DATA_BLOCK DB_AIS
TITLE = Analog Inputs SRC
//Analog Input Source DATA Block
VERSION : 0.1
  STRUCT
K04HJA10CR001XQ01 : UAI_SRC; //HOØÁK È.1 - VELIKOST PLAMENE 4-20mA
K04HJA20CR001XQ01 : UAI_SRC; //HOØÁK È.2 - VELIKOST PLAMENE 4-20mA
K04HJA30CR001XQ01 : UAI_SRC; //HOØÁK È.3 - VELIKOST PLAMENE 4-20mA
K04HJA40CR001XQ01 : UAI_SRC; //HOØÁK È.4 - VELIKOST PLAMENE 4-20mA
K04HHG36AS001XQ01 : UAI_SRC; //HOØÁK È.1 - POLOHA KLAPKY PLYNU
K04HHL11AS010XQ01 : UAI_SRC; //HOØÁK È.1 - POLOHA KLAPKY VZDUCHU
K04HHG37AS001XQ01 : UAI_SRC; //HOØÁK È.2 - POLOHA KLAPKY PLYNU
K04HHL71AS010XQ01 : UAI_SRC; //HOØÁK È.2 - POLOHA KLAPKY VZDUCHU
K04HHG38AS001XQ01 : UAI_SRC; //HOØÁK È.3 - POLOHA KLAPKY PLYNU
K04HHL51AS010XQ01 : UAI_SRC; //HOØÁK È.3 - POLOHA KLAPKY VZDUCHU
K04HHG39AS001XQ01 : UAI_SRC; //HOØÁK È.4 - POLOHA KLAPKY PLYNU
K04HHL31AS010XQ01 : UAI_SRC; //HOØÁK È.4 - POLOHA KLAPKY VZDUCHU
PIW536 : UAI_SRC; //REZERVA
PIW538 : UAI_SRC; //REZERVA
PIW540 : UAI_SRC; //REZERVA
PIW542 : UAI_SRC; //REZERVA
END_STRUCT ;
BEGIN

K04HJA10CR001XQ01.cMEAS_TYPE := 00;
K04HJA10CR001XQ01.cENABLE_REV := FALSE;
K04HJA10CR001XQ01.cLRANGE := 0.000;
K04HJA10CR001XQ01.cHRANGE := 100.000;
K04HJA10CR001XQ01.cENABLE_SQRT := FALSE;
K04HJA10CR001XQ01.cENABLE_LOLO := False;
K04HJA10CR001XQ01.cENABLE_LO := False;
K04HJA10CR001XQ01.cENABLE_HIHI := False;
K04HJA10CR001XQ01.cENABLE_HI := False;
K04HJA10CR001XQ01.cSET_LOLO := 0.000;
K04HJA10CR001XQ01.cSET_LO := 0.000;
K04HJA10CR001XQ01.cSET_HIHI := 100.000;
K04HJA10CR001XQ01.cSET_HI := 100.000;
K04HJA20CR001XQ01.cMEAS_TYPE := 00;
K04HJA20CR001XQ01.cENABLE_REV := FALSE;
K04HJA20CR001XQ01.cLRANGE := 0.000;
K04HJA20CR001XQ01.cHRANGE := 100.000;
K04HJA20CR001XQ01.cENABLE_SQRT := FALSE;
K04HJA20CR001XQ01.cENABLE_LOLO := False;
K04HJA20CR001XQ01.cENABLE_LO := False;
K04HJA20CR001XQ01.cENABLE_HIHI := False;
K04HJA20CR001XQ01.cENABLE_HI := False;
K04HJA20CR001XQ01.cSET_LOLO := 0.000;
K04HJA20CR001XQ01.cSET_LO := 0.000;
K04HJA20CR001XQ01.cSET_HIHI := 100.000;
K04HJA20CR001XQ01.cSET_HI := 100.000;
K04HJA30CR001XQ01.cMEAS_TYPE := 00;
K04HJA30CR001XQ01.cENABLE_REV := FALSE;
K04HJA30CR001XQ01.cLRANGE := 0.000;
K04HJA30CR001XQ01.cHRANGE := 100.000;
K04HJA30CR001XQ01.cENABLE_SQRT := FALSE;
K04HJA30CR001XQ01.cENABLE_LOLO := False;
K04HJA30CR001XQ01.cENABLE_LO := False;
K04HJA30CR001XQ01.cENABLE_HIHI := False;
K04HJA30CR001XQ01.cENABLE_HI := False;
K04HJA30CR001XQ01.cSET_LOLO := 0.000;
K04HJA30CR001XQ01.cSET_LO := 0.000;
K04HJA30CR001XQ01.cSET_HIHI := 100.000;
K04HJA30CR001XQ01.cSET_HI := 100.000;
K04HJA40CR001XQ01.cMEAS_TYPE := 00;
K04HJA40CR001XQ01.cENABLE_REV := FALSE;
K04HJA40CR001XQ01.cLRANGE := 0.000;
K04HJA40CR001XQ01.cHRANGE := 100.000;
K04HJA40CR001XQ01.cENABLE_SQRT := FALSE;
K04HJA40CR001XQ01.cENABLE_LOLO := False;
K04HJA40CR001XQ01.cENABLE_LO := False;
K04HJA40CR001XQ01.cENABLE_HIHI := False;
K04HJA40CR001XQ01.cENABLE_HI := False;
K04HJA40CR001XQ01.cSET_LOLO := 0.000;
K04HJA40CR001XQ01.cSET_LO := 0.000;
K04HJA40CR001XQ01.cSET_HIHI := 100.000;
K04HJA40CR001XQ01.cSET_HI := 100.000;
K04HHG36AS001XQ01.cMEAS_TYPE := 00;
K04HHG36AS001XQ01.cENABLE_REV := FALSE;
K04HHG36AS001XQ01.cLRANGE := 0.000;
K04HHG36AS001XQ01.cHRANGE := 100.000;
K04HHG36AS001XQ01.cENABLE_SQRT := FALSE;
K04HHG36AS001XQ01.cENABLE_LOLO := False;
K04HHG36AS001XQ01.cENABLE_LO := False;
K04HHG36AS001XQ01.cENABLE_HIHI := False;
K04HHG36AS001XQ01.cENABLE_HI := False;
K04HHG36AS001XQ01.cSET_LOLO := 0.000;
K04HHG36AS001XQ01.cSET_LO := 0.000;
K04HHG36AS001XQ01.cSET_HIHI := 100.000;
K04HHG36AS001XQ01.cSET_HI := 100.000;
K04HHL11AS010XQ01.cMEAS_TYPE := 00;
K04HHL11AS010XQ01.cENABLE_REV := FALSE;
K04HHL11AS010XQ01.cLRANGE := 0.000;
K04HHL11AS010XQ01.cHRANGE := 100.000;
K04HHL11AS010XQ01.cENABLE_SQRT := FALSE;
K04HHL11AS010XQ01.cENABLE_LOLO := False;
K04HHL11AS010XQ01.cENABLE_LO := False;
K04HHL11AS010XQ01.cENABLE_HIHI := False;
K04HHL11AS010XQ01.cENABLE_HI := False;
K04HHL11AS010XQ01.cSET_LOLO := 0.000;
K04HHL11AS010XQ01.cSET_LO := 0.000;
K04HHL11AS010XQ01.cSET_HIHI := 100.000;
K04HHL11AS010XQ01.cSET_HI := 100.000;
K04HHG37AS001XQ01.cMEAS_TYPE := 00;
K04HHG37AS001XQ01.cENABLE_REV := FALSE;
K04HHG37AS001XQ01.cLRANGE := 0.000;
K04HHG37AS001XQ01.cHRANGE := 100.000;
K04HHG37AS001XQ01.cENABLE_SQRT := FALSE;
K04HHG37AS001XQ01.cENABLE_LOLO := False;
K04HHG37AS001XQ01.cENABLE_LO := False;
K04HHG37AS001XQ01.cENABLE_HIHI := False;
K04HHG37AS001XQ01.cENABLE_HI := False;
K04HHG37AS001XQ01.cSET_LOLO := 0.000;
K04HHG37AS001XQ01.cSET_LO := 0.000;
K04HHG37AS001XQ01.cSET_HIHI := 100.000;
K04HHG37AS001XQ01.cSET_HI := 100.000;
K04HHL71AS010XQ01.cMEAS_TYPE := 00;
K04HHL71AS010XQ01.cENABLE_REV := FALSE;
K04HHL71AS010XQ01.cLRANGE := 0.000;
K04HHL71AS010XQ01.cHRANGE := 100.000;
K04HHL71AS010XQ01.cENABLE_SQRT := FALSE;
K04HHL71AS010XQ01.cENABLE_LOLO := False;
K04HHL71AS010XQ01.cENABLE_LO := False;
K04HHL71AS010XQ01.cENABLE_HIHI := False;
K04HHL71AS010XQ01.cENABLE_HI := False;
K04HHL71AS010XQ01.cSET_LOLO := 0.000;
K04HHL71AS010XQ01.cSET_LO := 0.000;
K04HHL71AS010XQ01.cSET_HIHI := 100.000;
K04HHL71AS010XQ01.cSET_HI := 100.000;
K04HHG38AS001XQ01.cMEAS_TYPE := 00;
K04HHG38AS001XQ01.cENABLE_REV := FALSE;
K04HHG38AS001XQ01.cLRANGE := 0.000;
K04HHG38AS001XQ01.cHRANGE := 100.000;
K04HHG38AS001XQ01.cENABLE_SQRT := FALSE;
K04HHG38AS001XQ01.cENABLE_LOLO := False;
K04HHG38AS001XQ01.cENABLE_LO := False;
K04HHG38AS001XQ01.cENABLE_HIHI := False;
K04HHG38AS001XQ01.cENABLE_HI := False;
K04HHG38AS001XQ01.cSET_LOLO := 0.000;
K04HHG38AS001XQ01.cSET_LO := 0.000;
K04HHG38AS001XQ01.cSET_HIHI := 100.000;
K04HHG38AS001XQ01.cSET_HI := 100.000;
K04HHL51AS010XQ01.cMEAS_TYPE := 00;
K04HHL51AS010XQ01.cENABLE_REV := FALSE;
K04HHL51AS010XQ01.cLRANGE := 0.000;
K04HHL51AS010XQ01.cHRANGE := 100.000;
K04HHL51AS010XQ01.cENABLE_SQRT := FALSE;
K04HHL51AS010XQ01.cENABLE_LOLO := False;
K04HHL51AS010XQ01.cENABLE_LO := False;
K04HHL51AS010XQ01.cENABLE_HIHI := False;
K04HHL51AS010XQ01.cENABLE_HI := False;
K04HHL51AS010XQ01.cSET_LOLO := 0.000;
K04HHL51AS010XQ01.cSET_LO := 0.000;
K04HHL51AS010XQ01.cSET_HIHI := 100.000;
K04HHL51AS010XQ01.cSET_HI := 100.000;
K04HHG39AS001XQ01.cMEAS_TYPE := 00;
K04HHG39AS001XQ01.cENABLE_REV := FALSE;
K04HHG39AS001XQ01.cLRANGE := 0.000;
K04HHG39AS001XQ01.cHRANGE := 100.000;
K04HHG39AS001XQ01.cENABLE_SQRT := FALSE;
K04HHG39AS001XQ01.cENABLE_LOLO := False;
K04HHG39AS001XQ01.cENABLE_LO := False;
K04HHG39AS001XQ01.cENABLE_HIHI := False;
K04HHG39AS001XQ01.cENABLE_HI := False;
K04HHG39AS001XQ01.cSET_LOLO := 0.000;
K04HHG39AS001XQ01.cSET_LO := 0.000;
K04HHG39AS001XQ01.cSET_HIHI := 100.000;
K04HHG39AS001XQ01.cSET_HI := 100.000;
K04HHL31AS010XQ01.cMEAS_TYPE := 00;
K04HHL31AS010XQ01.cENABLE_REV := FALSE;
K04HHL31AS010XQ01.cLRANGE := 0.000;
K04HHL31AS010XQ01.cHRANGE := 100.000;
K04HHL31AS010XQ01.cENABLE_SQRT := FALSE;
K04HHL31AS010XQ01.cENABLE_LOLO := False;
K04HHL31AS010XQ01.cENABLE_LO := False;
K04HHL31AS010XQ01.cENABLE_HIHI := False;
K04HHL31AS010XQ01.cENABLE_HI := False;
K04HHL31AS010XQ01.cSET_LOLO := 0.000;
K04HHL31AS010XQ01.cSET_LO := 0.000;
K04HHL31AS010XQ01.cSET_HIHI := 100.000;
K04HHL31AS010XQ01.cSET_HI := 100.000;
PIW536.cMEAS_TYPE := 00;
PIW536.cENABLE_REV := FALSE;
PIW536.cLRANGE := 0.000;
PIW536.cHRANGE := 100.000;
PIW536.cENABLE_SQRT := FALSE;
PIW536.cENABLE_LOLO := False;
PIW536.cENABLE_LO := False;
PIW536.cENABLE_HIHI := False;
PIW536.cENABLE_HI := False;
PIW536.cSET_LOLO := 0.000;
PIW536.cSET_LO := 0.000;
PIW536.cSET_HIHI := 100.000;
PIW536.cSET_HI := 100.000;
PIW538.cMEAS_TYPE := 00;
PIW538.cENABLE_REV := FALSE;
PIW538.cLRANGE := 0.000;
PIW538.cHRANGE := 100.000;
PIW538.cENABLE_SQRT := FALSE;
PIW538.cENABLE_LOLO := False;
PIW538.cENABLE_LO := False;
PIW538.cENABLE_HIHI := False;
PIW538.cENABLE_HI := False;
PIW538.cSET_LOLO := 0.000;
PIW538.cSET_LO := 0.000;
PIW538.cSET_HIHI := 100.000;
PIW538.cSET_HI := 100.000;
PIW540.cMEAS_TYPE := 00;
PIW540.cENABLE_REV := FALSE;
PIW540.cLRANGE := 0.000;
PIW540.cHRANGE := 100.000;
PIW540.cENABLE_SQRT := FALSE;
PIW540.cENABLE_LOLO := False;
PIW540.cENABLE_LO := False;
PIW540.cENABLE_HIHI := False;
PIW540.cENABLE_HI := False;
PIW540.cSET_LOLO := 0.000;
PIW540.cSET_LO := 0.000;
PIW540.cSET_HIHI := 100.000;
PIW540.cSET_HI := 100.000;
PIW542.cMEAS_TYPE := 00;
PIW542.cENABLE_REV := FALSE;
PIW542.cLRANGE := 0.000;
PIW542.cHRANGE := 100.000;
PIW542.cENABLE_SQRT := FALSE;
PIW542.cENABLE_LOLO := False;
PIW542.cENABLE_LO := False;
PIW542.cENABLE_HIHI := False;
PIW542.cENABLE_HI := False;
PIW542.cSET_LOLO := 0.000;
PIW542.cSET_LO := 0.000;
PIW542.cSET_HIHI := 100.000;
PIW542.cSET_HI := 100.000;
END_DATA_BLOCK
